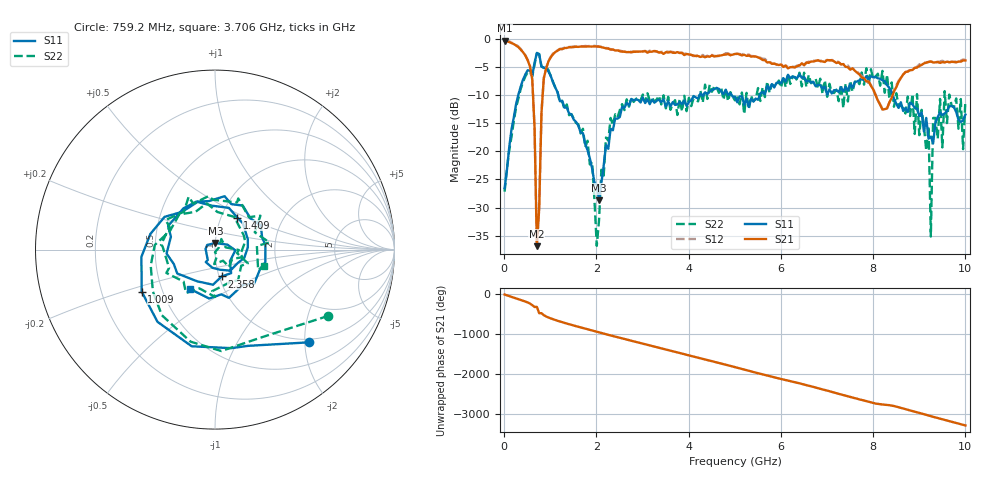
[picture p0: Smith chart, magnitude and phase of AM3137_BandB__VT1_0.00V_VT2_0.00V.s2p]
! Date/Time: Tue, Nov 13, 2018 4:51 PM
! Network Analyzer: Agilent Technologies E8364B Rev: A.07.50.67
! Sweep from 0.010 to 10.000 GHz, 201 Points, Sweep Type: LIN
! Power Supply: -0.000 V, 0.000 A
# Hz S DB R 50
!freq MagS11 AngS11 MagS21 AngS21 MagS12 AngS12 MagS22 AngS22
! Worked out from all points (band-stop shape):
!   201 points, 10 MHz to 10 GHz, reference 50 ohm
!   highest |S21| = -0.30 dB at 10 MHz (marker M1); lowest = -36.9 dB at 709.3 MHz (marker M2)
!   |S21| within 3 dB of the highest: start of sweep to 481.4 MHz; 1.007 GHz to 5.516 GHz (4.51 GHz wide, 138 % of centre)
!   lowest |S11| = -28.7 dB at 2.058 GHz (marker M3), VSWR 1.08, Z = 50 + j3.67 ohm
!   |S11| at or under -10 dB: 1.175 GHz to 4.238 GHz (3.064 GHz wide, 113 % of centre); 4.934 GHz to 5.541 GHz (606.3 MHz wide, 11.6 % of centre); 8.424 GHz to end of sweep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
!   |S22| runs from -36.8 to -2.6 dB; largest |S21 - S12| = 0.032
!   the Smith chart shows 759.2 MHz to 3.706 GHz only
!   S11 on the Smith chart (normalised r, x): 759.2 MHz: 0.93, -2.09; 1.009 GHz: 0.38, -0.23; 1.409 GHz: 1.19, +0.45; 2.358 GHz: 1.03, -0.32; 3.706 GHz: 0.69, -0.33
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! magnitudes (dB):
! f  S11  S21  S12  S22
! 10 MHz  -26.6  -0.3  -0.3  -27.2
! 609.4 MHz  -6.5  -7.2  -7.2  -6.7
! 709.3 MHz  -2.5  -36.9  -36.4  -2.6
! 759.2 MHz  -2.7  -30.2  -30.0  -2.7
! 859.2 MHz  -5.1  -7.0  -6.9  -5.2
! 1.009 GHz  -6.5  -3.3  -3.2  -6.5
! 1.409 GHz  -13.3  -1.5  -1.4  -13.6
! 1.708 GHz  -16.8  -1.3  -1.3  -16.0
! 2.008 GHz  -25.9  -1.3  -1.3  -36.8
! 2.058 GHz  -28.7  -1.4  -1.3  -32.2
! 2.358 GHz  -16.2  -1.9  -1.9  -15.3
! 3.357 GHz  -10.8  -2.4  -2.4  -10.1
! 3.706 GHz  -11.7  -2.5  -2.4  -10.9
! 5.005 GHz  -10.3  -2.7  -2.7  -10.9
! 6.703 GHz  -7.6  -4.0  -3.8  -7.6
! 8.352 GHz  -8.7  -11.3  -11.3  -10.7
! 9.201 GHz  -17.7  -4.1  -4.1  -15.5
! 9.251 GHz  -17.4  -4.0  -4.0  -35.2
! 9.301 GHz  -18.6  -4.2  -4.1  -14.1
! 9.9 GHz  -14.8  -4.0  -3.8  -10.7
! 9.95 GHz  -14.5  -3.8  -3.6  -19.6
! 10 GHz  -13.5  -3.8  -3.7  -10.9
